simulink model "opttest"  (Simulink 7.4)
settings: Solver=ode45  StartTime=0.0  StopTime=30  RelTol=1e-3
undefined symbols (not defined in the file or in its folder): L2, Norm
libraries: RCTblocks x2, RCTWCSIMLib x2

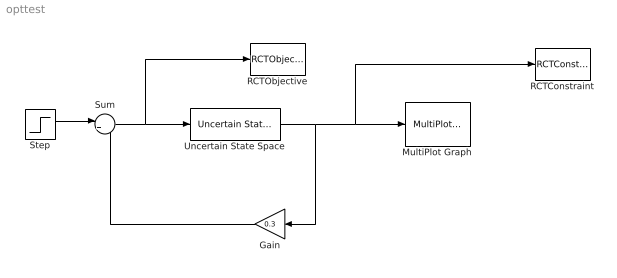
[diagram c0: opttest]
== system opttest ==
  Gain : Gain  Gain=0.3  ParameterDataType=sfix(16)  ParameterScaling=2^0  OutDataType=sfix(16)  OutScaling=2^0
  MultiPlot Graph : RCTblocks/MultiPlot Graph  Tag=MultiPlot  SystemSampleTime=-1  tmin=0  tmax=20  ymin=-1  ymax=1  Tsamp=-1  vnamesave=multisimout
  RCTConstraint : RCTWCSIMLib/RCTConstraint  Tag=WCSIMConstraint  SystemSampleTime=-1  ConType=Pointwise Maximum  ConMfile=''  ConUB=0.9  ConLB=-inf  VarName=WCSIMConstraint  DataPts=inf  SampleTime=-1  SaveFormat=Structure With Time  LogFixedPoint=off
  RCTObjective : RCTWCSIMLib/RCTObjective  Tag=WCSIMObjective  SystemSampleTime=-1  ObjType=L2 Norm  MaxMin=Minimize  ObjMfile=''  VarName=WCSIMObjective  DataPts=inf  SampleTime=-1  SaveFormat=Structure With Time  LogFixedPoint=off
  Step : Step  SampleTime=0
  Sum : Sum  Inputs=|+-  OutDataType=sfix(16)  OutScaling=2^0
  Uncertain State Space : RCTblocks/Uncertain State Space  Tag=USS  SystemSampleTime=-1  USystem=G  UValue=GUncValue  X0=[0]  uX0=[]
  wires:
  Uncertain State Space/1 -> Gain/1, MultiPlot Graph/1, RCTConstraint/1
  Step/1 -> Sum/1
  Sum/1 -> RCTObjective/1, Uncertain State Space/1
  Gain/1 -> Sum/2
